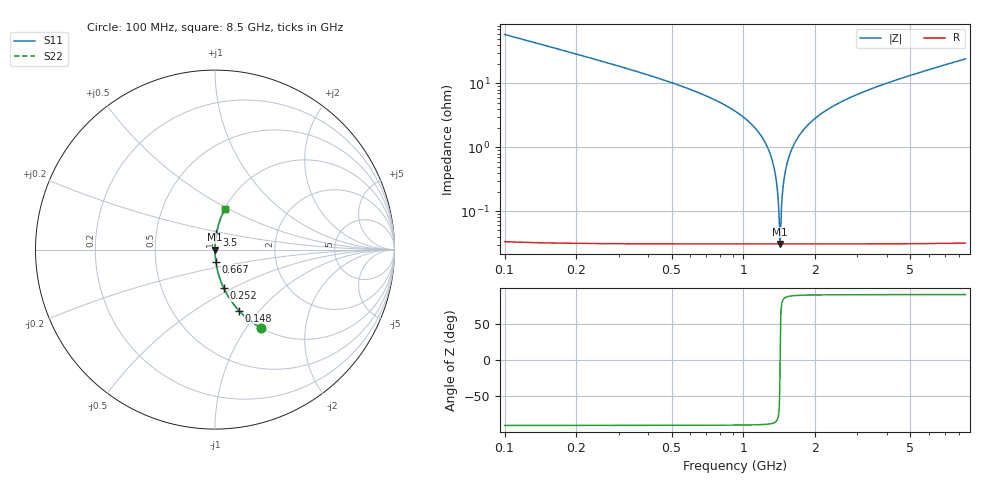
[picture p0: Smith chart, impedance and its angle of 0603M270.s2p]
! Created Wed Apr 18 16:46:32 2012
# hz S ma R 50
! 2 Port Network Data from SP1.SP block
! freq  magS11  angS11  magS21  angS21  magS12  angS12  magS22  angS22
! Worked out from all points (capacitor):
!   8401 points, 100 MHz to 8.5 GHz, reference 50 ohm
!   read as one part in series: C = 27.1 pF near 142 MHz
!   lowest |Z| = 30.8 mohm at 1.424 GHz (marker M1)
!   series resonance near 1.424 GHz, so ESL is about 460 pH
!   S11 on the Smith chart (normalised r, x): 100 MHz: 1.00, -1.17; 148 MHz: 1.00, -0.79; 252 MHz: 1.00, -0.45; 667 MHz: 1.00, -0.14; 3.5 GHz: 1.00, +0.17; 8.5 GHz: 1.00, +0.49
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1e8  0.5044 -59.7  0.8632 30.3  0.8632 30.3  0.5044 -59.7
1.48e8  0.3653 -68.5  0.9306 21.4  0.9306 21.4  0.3653 -68.5
2.52e8  0.2201 -77.2  0.9752 12.7  0.9752 12.7  0.2201 -77.2
6.67e8  0.06855 -85.8  0.9973 3.9  0.9973 3.9  0.06855 -85.8
1.02e9  0.02801 -87.8  0.9993 1.6  0.9993 1.6  0.02801 -87.8
1.222e9  0.01266 -87.9  0.9996 0.7  0.9996 0.7  0.01266 -87.9
1.332e9  0.005508 -86.5  0.9997 0.3  0.9997 0.3  0.005508 -86.5
1.364e9  0.003551 -84.8  0.9997 0.2  0.9997 0.2  0.003551 -84.8
1.397e9  0.001594 -78.8  0.9997 0.1  0.9997 0.1  0.001594 -78.8
1.424e9  0.0003083 2.8  0.9997 -0.0  0.9997 -0.0  0.0003083 2.8
1.451e9  0.001595 78.8  0.9997 -0.1  0.9997 -0.1  0.001595 78.8
1.5e9  0.004318 85.7  0.9997 -0.2  0.9997 -0.2  0.004318 85.7
1.554e9  0.007239 87.1  0.9997 -0.4  0.9997 -0.4  0.007239 87.1
1.633e9  0.01135 87.8  0.9996 -0.7  0.9996 -0.7  0.01135 87.8
1.881e9  0.02328 87.9  0.9994 -1.3  0.9994 -1.3  0.02328 87.9
2.288e9  0.04061 87.2  0.9989 -2.3  0.9989 -2.3  0.04061 87.2
2.9e9  0.06371 86.1  0.9977 -3.7  0.9977 -3.7  0.06371 86.1
3.5e9  0.08447 84.9  0.9961 -4.8  0.9961 -4.8  0.08447 84.9
4.3e9  0.1106 83.5  0.9936 -6.3  0.9936 -6.3  0.1106 83.5
5.7e9  0.1538 81.0  0.9878 -8.8  0.9878 -8.8  0.1538 81.0
7.1e9  0.1953 78.6  0.9804 -11.3  0.9804 -11.3  0.1953 78.6
8.5e9  0.2357 76.3  0.9715 -13.6  0.9715 -13.6  0.2357 76.3
